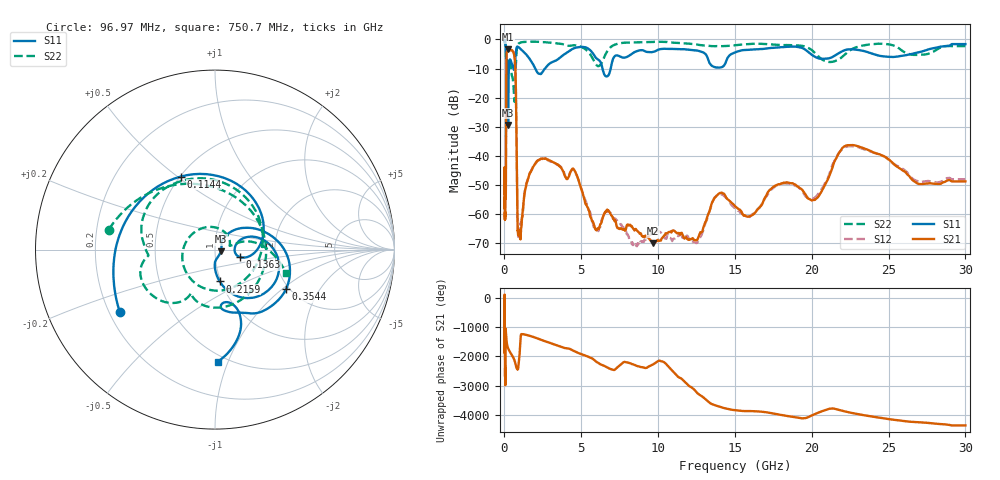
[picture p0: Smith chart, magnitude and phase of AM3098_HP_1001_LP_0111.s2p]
! Date/Time: Thu, Feb 28, 2019 8:41 AM
! Network Analyzer: Agilent Technologies E8364B Rev: A.07.50.67
! Sweep from 0.010 to 30.000 GHz, 1601 Points, Sweep Type: LOG
! Power Supply: 5.023 V, 0.002 A
# Hz S DB R 50
!freq MagS11 AngS11 MagS21 AngS21 MagS12 AngS12 MagS22 AngS22
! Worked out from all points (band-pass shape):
!   1601 points, 10 MHz to 30 GHz, reference 50 ohm
!   highest |S21| = -3.43 dB at 236.3 MHz (marker M1); lowest = -70.2 dB at 9.682 GHz (marker M2)
!   |S21| within 3 dB of the highest: 129.4 MHz to 664.5 MHz (535.1 MHz wide, 135 % of centre)
!   lowest |S11| = -29.4 dB at 237.5 MHz (marker M3), VSWR 1.07, Z = 53.4 - j0.934 ohm
!   |S11| at or under -10 dB: 199.1 MHz to 287.6 MHz (88.57 MHz wide, 36.4 % of centre); 2.008 GHz to 2.645 GHz (636.6 MHz wide, 27.4 % of centre); 6.379 GHz to 6.915 GHz (535.6 MHz wide, 8.06 % of centre)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
!   |S22| runs from -21.5 to -0.5 dB; largest |S21 - S12| = 0.0092
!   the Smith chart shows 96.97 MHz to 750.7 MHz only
!   S11 on the Smith chart (normalised r, x): 96.97 MHz: 0.24, -0.28; 114.4 MHz: 0.50, +0.51; 136.3 MHz: 1.32, -0.11; 215.9 MHz: 0.99, -0.36; 354.4 MHz: 1.92, -1.07; 750.7 MHz: 0.45, -0.92
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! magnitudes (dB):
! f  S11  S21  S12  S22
! 10 MHz  -0.3  -44.4  -46.4  -0.5
! 38.04 MHz  -0.5  -59.7  -59.2  -0.9
! 87.73 MHz  -2.7  -52.7  -56.4  -2.9
! 96.97 MHz  -4.0  -43.6  -44.3  -4.4
! 114.4 MHz  -6.9  -16.7  -16.7  -10.8
! 136.3 MHz  -16.7  -5.2  -5.1  -11.1
! 144.7 MHz  -19.0  -4.5  -4.5  -10.7
! 215.9 MHz  -14.9  -3.6  -3.5  -8.2
! 236.3 MHz  -29.3  -3.4  -3.4  -8.6
! 237.5 MHz  -29.4  -3.4  -3.4  -8.6
! 354.4 MHz  -6.9  -3.8  -3.8  -7.4
! 550.5 MHz  -9.4  -4.1  -4.1  -13.8
! 662.4 MHz  -9.5  -6.3  -6.3  -21.5
! 750.7 MHz  -4.1  -19.6  -19.6  -7.6
! 898.9 MHz  -2.6  -67.0  -68.0  -1.5
! 2.084 GHz  -10.8  -42.1  -42.3  -0.8
! 4.503 GHz  -3.1  -44.6  -45.0  -2.0
! 7.926 GHz  -6.1  -64.8  -66.2  -1.1
! 9.682 GHz  -4.3  -70.2  -66.5  -0.9
! 20.2 GHz  -5.9  -55.2  -54.4  -4.6
! 22.67 GHz  -3.4  -36.3  -36.8  -3.2
! 30 GHz  -1.6  -48.8  -48.1  -2.3
